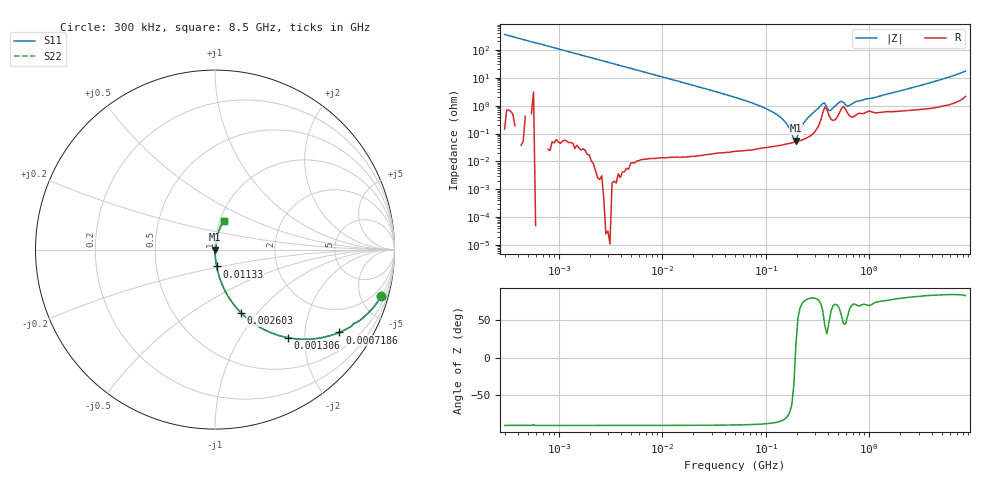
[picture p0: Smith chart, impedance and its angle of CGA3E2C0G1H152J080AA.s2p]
! S-parameter Generated by TDK Corporation
! Copyright(C) 2015 TDK Corporation.
! All Rights Reserved.
! TDK P/N: CGA3E2C0G1H152J080AA (Multilayer Ceramic Chip Capacitors)
! Property: C=1.5nF
! Size(LxWxT): 1.6x0.8x0.8mm, 0.063x0.031x0.031inches
! Model Type: s2p (Touchstone File Format Version 1.0)
! Frequency: DC=Yes Start=0.3MHz Stop=8500MHz 225points Log-sweep
! Note:
! Model Generated on Jun. 23, 2015
! Hash(MD5):
! Port Assignments:
!  1 ---| |--- 2
! Applicable Conditions:
!  Temperature = 25 degC
!  DC Bias Voltage = 0 V
!  Small Signal Operation
! Terms and conditions regarding TDK Simulation Models
! (1)This simulation model is being provided solely for informational purposes. Please refer to the specifications of the products in terms of detailed characteristics of such products.
! (2)In no event shall TDK Corporation of any of its subsidiaries be liable for any loss or damage arising, directly or indirectly,
!  From any information contained in this simulation model, including, but not limited to loss or damages arising from any inaccuracies, omissions or errors in connection with such information.
! (3)Any and all copyrights on this simulation model are owned by TDK Corporation.
!  Duplication or redistribution of this simulation model without prior written permission from TDK Corporation is prohibited.
! (4)This simulation model is subject to any modification or change without any prior notice.
! (5)Neither TDK Corporation nor any of its subsidiaries shall make any warranty, express or implied,
!  Including but not limited to the correctness, implied warranties of merchantability and fitness for a particular purpose with respect to this simulation models.
! (6)The use of this simulation model shall be deemed to have consented to the terms and conditions hereof.
# MHz S MA R 50
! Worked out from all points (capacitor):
!   224 points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, 300 kHz to 8.5 GHz, reference 50 ohm
!   read as one part in series: C = 1.49 nF near 314.1 kHz
!   lowest |Z| = 55.5 mohm at 196 MHz (marker M1)
!   series resonance near 193 MHz, so ESL is about 460 pH
!   S11 on the Smith chart (normalised r, x): 300 kHz: 1.00, -7.15; 718.6 kHz: 1.00, -3.00; 1.306 MHz: 1.00, -1.65; 2.603 MHz: 1.00, -0.83; 11.33 MHz: 1.00, -0.19; 8.5 GHz: 1.04, +0.34
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0.3  0.9629 -15.6  0.2695 74.3  0.2695 74.3  0.9629 -15.6
0.7185633  0.8322 -33.7  0.5544 56.3  0.5544 56.3  0.8322 -33.7
1.306219  0.6362 -50.5  0.7712 39.5  0.7712 39.5  0.6362 -50.5
1.72111  0.5306 -57.9  0.8474 32.0  0.8474 32.0  0.5306 -57.9
2.603142  0.3826 -67.5  0.9239 22.5  0.9239 22.5  0.3826 -67.5
9.430415  0.1134 -83.4  0.9934 6.5  0.9934 6.5  0.1134 -83.4
11.33425  0.09443 -84.5  0.9954 5.4  0.9954 5.4  0.09443 -84.5
51.67171  0.0194 -88.2  0.9996 1.1  0.9996 1.1  0.0194 -88.2
129.5872  0.004647 -85.3  0.9996 0.3  0.9996 0.3  0.004647 -85.3
163.0757  0.001986 -77.4  0.9996 0.1  0.9996 0.1  0.001986 -77.4
187.1913  0.0005998 -35.4  0.9995 0.0  0.9995 0.0  0.0005998 -35.4
195.9978  0.0005528 18.6  0.9995 -0.0  0.9995 -0.0  0.0005528 18.6
224.9819  0.001951 72.4  0.9994 -0.1  0.9994 -0.1  0.001951 72.4
283.1228  0.005268 79.4  0.999 -0.3  0.999 -0.3  0.005268 79.4
356.2888  0.01196 61.6  0.9944 -0.6  0.9944 -0.6  0.01196 61.6
373.0505  0.01211 41.8  0.991 -0.5  0.991 -0.5  0.01211 41.8
408.9767  0.006535 47.0  0.9956 -0.3  0.9956 -0.3  0.006535 47.0
538.8791  0.01427 55.8  0.9921 -0.7  0.9921 -0.7  0.01427 55.8
618.5683  0.009519 55.1  0.9946 -0.4  0.9946 -0.4  0.009519 55.1
743.4462  0.01391 70.1  0.9953 -0.8  0.9953 -0.8  0.01391 70.1
1551.304  0.0265 75.3  0.9936 -1.5  0.9936 -1.5  0.0265 75.3
8500  0.1665 73.4  0.9656 -9.5  0.9656 -9.5  0.1665 73.4
